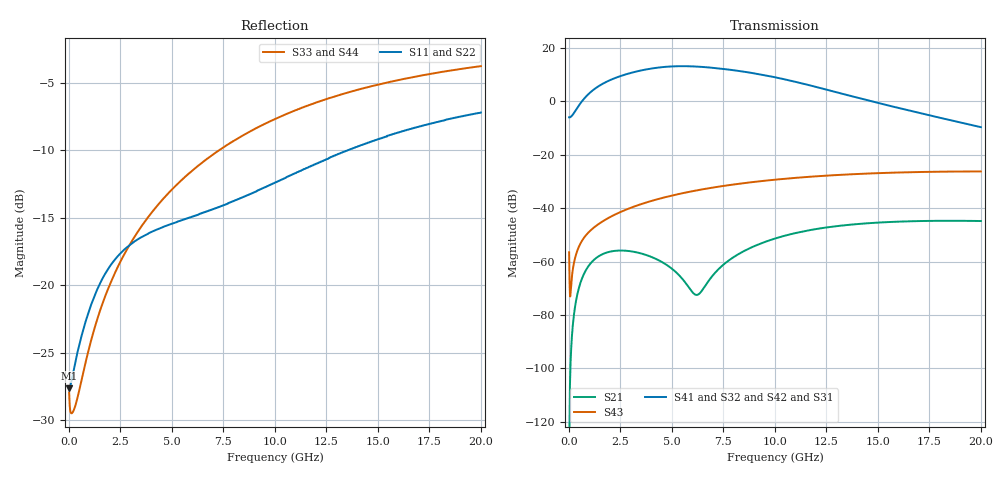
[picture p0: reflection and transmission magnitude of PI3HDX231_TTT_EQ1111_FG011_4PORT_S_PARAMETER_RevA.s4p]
! NPort=4 DATA=2000 NOISE=0 GROUPDELAY=0 COMPLEX_DATAFORMAT=POLAR
! NumOfBlock=1 NumOfParam=0
! .MODEL Smodel S TSTONEFILE=PI3HDX231_TTT_EQ1111_FG011_4PORT_S_PARAMETER_RevA.s4p TYPE=S
!  -- The above .MODEL line can be used for the S element in the netlist.
! The s parameter is extracted from the linear redriver, it is not bi-directional; only s(4,1)s(4,2) and s(3,1)s(3,2)
! should be the insertion loss
!Port definition:
!Port1 = input+
!Port2 = input-
!Port3 = output+
!Port4 = output-
# Hz S MA R  50
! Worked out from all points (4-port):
!   2000 points, 10 MHz to 20 GHz, reference 50 ohm
!   strongest paths, dB at 10 MHz, 5.01 GHz, 10.01 GHz, 15.01 GHz, 20 GHz:
!     S41: -5.9, 13.1, 9.0, -0.6, -9.6
!     S32: -5.9, 13.1, 9.0, -0.5, -9.5
!     S42: -5.9, 13.1, 8.9, -0.7, -9.8
!     S31: -5.9, 13.0, 8.8, -0.9, -10.0
!     S43: -56.5, -35.2, -29.3, -26.8, -26.2
!     S21: -134.8, -62.7, -51.3, -45.4, -44.8
!   lowest |S11| = -27.6 dB at 10 MHz (marker M1), VSWR 1.09, Z = 46 - j0.0776 ohm
!   |S11| at or under -10 dB: start of sweep to 13.55 GHz
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1e7  0.04152 -178.8  1.825e-07 -13.9  0 0.0  0 0.0
     1.825e-07 -14.0  0.04152 -178.8  0 0.0  0 0.0
     0.5043 0.5  0.5043 -179.5  0.04012 -3.2  0.0015 -70.3
     0.5043 -179.5  0.5043 0.5  0.0015 -70.3  0.04012 -3.2
3.17e9  0.145 -140.7  0.001526 12.3  4.787e-11 -117.9  3.947e-11 -109.8
        0.001527 12.3  0.145 -140.8  3.854e-11 -110.3  4.916e-11 -117.2
        3.521 -26.1  3.532 153.7  0.1505 -96.1  0.0108 70.3
        3.554 153.9  3.539 -25.5  0.01079 70.2  0.1505 -96.1
5.21e9  0.1712 -139.7  0.0006251 -11.6  9.084e-10 176.0  6.264e-10 -161.6
        0.0006287 -11.5  0.1711 -139.9  6.072e-10 -161.2  9.422e-10 175.9
        4.505 -91.9  4.526 88.0  0.2346 -103.1  0.01809 60.4
        4.561 87.9  4.543 -91.2  0.01804 60.3  0.2346 -103.1
7.42e9  0.1964 -134.9  0.0008319 103.4  6.951e-09 108.5  5.008e-09 140.3
        0.0008254 102.8  0.1959 -135.1  4.884e-09 141.7  7.195e-09 107.4
        4.023 -160.6  4.065 19.2  0.3209 -109.2  0.026 47.2
        4.096 18.9  4.066 -159.8  0.0259 47.2  0.321 -109.2
1.01e10  0.2413 -129.5  0.0028 84.4  3.427e-08 32.7  2.624e-08 64.3
         0.002783 84.2  0.24 -129.7  2.596e-08 66.1  3.505e-08 31.0
         2.716 125.7  2.775 -54.8  0.4152 -115.9  0.03467 29.9
         2.788 -55.4  2.754 126.6  0.03455 30.1  0.4153 -115.9
1.328e10  0.3098 -128.3  0.004789 50.9  1.069e-07 -42.9  8.37e-08 -16.9
          0.004759 50.7  0.3078 -128.3  8.412e-08 -15.2  1.078e-07 -44.7
          1.34 54.2  1.392 -127.1  0.5094 -123.0  0.04256 9.1
          1.391 -127.9  1.365 55.3  0.04248 9.4  0.5093 -123.1
2e10  0.4356 -135.6  0.005812 -3.9  3.73e-07 -162.9  2.784e-07 -146.1
      0.005768 -4.1  0.4339 -135.4  2.838e-07 -145.2  3.705e-07 -164.2
      0.3158 -51.5  0.3335 123.5  0.6464 -135.0  0.04885 -32.3
      0.33 122.9  0.3252 -50.4  0.04894 -32.1  0.6461 -135.0
